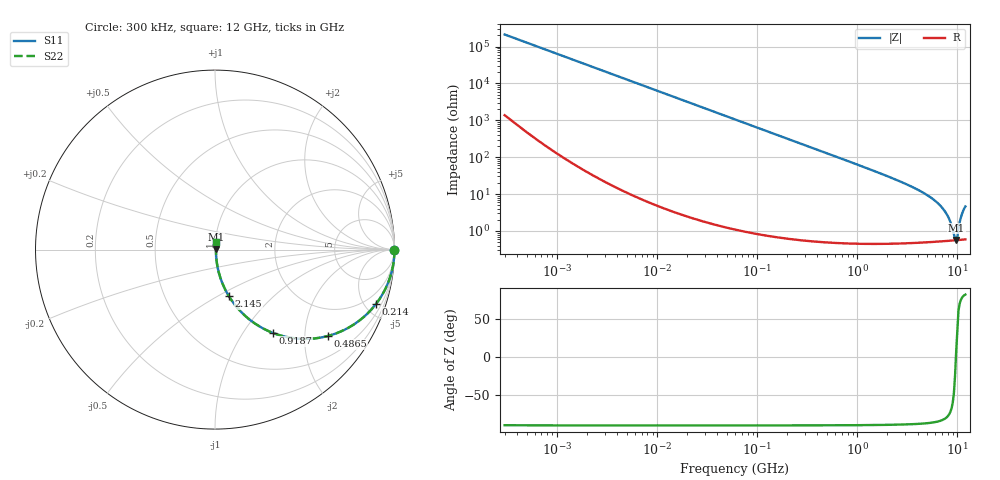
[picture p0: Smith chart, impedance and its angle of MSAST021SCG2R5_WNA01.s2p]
! MSAST021SCG2R5_WNA01  S-PARAMETER MODEL  ( General Type )
! Model Generated by TAIYO YUDEN Corporation (http://www.ty-top.com)
! Version 2.0
! TAIYO YUDEN Control No. 181101
! Copyright(c) 2015 TAIYO YUDEN CO.,LTD. All Rights Reserved.
! Product Description (link to TY-COMPAS)
! https://ds.yuden.co.jp/TYCOMPAS/or/detail?pn=MSAST021SCG2R5BWNA01&u=M
! Products Name : Multilayer Ceramic Capacitors
! Characteristics :
!  Capacitance : 2.5 pF , Rated Voltage : 25V , TCC : CG / C0G
!  Case Size : 0.25 x 0.125 / 0.0098 x 0.0049 [mm/inch] , Thickness : 0.125 / 0.0049 [mm/inch]
!  (Conditions: Temperature = 25 degC , DC Bias Current/Voltage = 0A / 0V)
! External Node Assignments :
!  1  o---| |---o  2
! GND o---------o GND
! Frequency Range : 0.3MHz  -  12000MHz  [ 401 STEP ]
# MHz S RI R 50
! Freq[MHz].  S11 Real  S11 Imag  S21 Real  S21 Imag  S12 Real  S12 Imag  S22 Real  S22 Imag
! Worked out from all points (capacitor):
!   401 points, 300 kHz to 12 GHz, reference 50 ohm
!   read as one part in series: C = 2.5 pF near 316.3 kHz
!   lowest |Z| = 566 mohm at 9.708 GHz (marker M1)
!   series resonance near 9.652 GHz, so ESL is about 110 pH
!   S11 on the Smith chart (normalised r, x): 300 kHz: open; 214 MHz: 1.01, -5.95; 486.5 MHz: 1.01, -2.61; 918.7 MHz: 1.01, -1.37; 2.145 GHz: 1.01, -0.56; 12 GHz: 1.01, +0.09
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0.3  1 -0.000471  3.28e-06 0.000471  3.28e-06 0.000471  1 -0.000471
1.769972  1 -0.00278  1.14e-05 0.00278  1.14e-05 0.00278  1 -0.00278
10.44266  0.9997 -0.0164  0.000281 0.0164  0.000281 0.0164  0.9997 -0.0164
60  0.9911 -0.0934  0.0089 0.0934  0.0089 0.0934  0.9911 -0.0934
213.9924  0.8979 -0.3018  0.1021 0.3018  0.1021 0.3018  0.8979 -0.3018
353.9943  0.7627 -0.424  0.2373 0.424  0.2373 0.424  0.7627 -0.424
486.4723  0.6297 -0.481  0.3703 0.481  0.3703 0.481  0.6297 -0.481
918.7169  0.3215 -0.4638  0.6785 0.4638  0.6785 0.4638  0.3215 -0.4638
1366.97  0.1748 -0.3749  0.8252 0.3749  0.8252 0.3749  0.1748 -0.3749
2088.533  0.0813 -0.2657  0.9187 0.2657  0.9187 0.2657  0.0813 -0.2657
2144.601  0.0773 -0.2592  0.9227 0.2592  0.9227 0.2592  0.0773 -0.2592
4050.141  0.021 -0.1261  0.979 0.1261  0.979 0.1261  0.021 -0.1261
6188.031  0.00868 -0.0597  0.9913 0.0597  0.9913 0.0597  0.00868 -0.0597
7064.448  0.00693 -0.0412  0.9931 0.0412  0.9931 0.0412  0.00693 -0.0412
7854.144  0.00606 -0.027  0.9939 0.027  0.9939 0.027  0.00606 -0.027
8503.825  0.00569 -0.0165  0.9943 0.0165  0.9943 0.0165  0.00569 -0.0165
9207.246  0.00555 -0.00603  0.9944 0.00603  0.9944 0.00603  0.00555 -0.00603
9454.42  0.00555 -0.00257  0.9944 0.00257  0.9944 0.00257  0.00555 -0.00257
9708.23  0.00558 0.000724  0.9944 -0.000724  0.9944 -0.000724  0.00558 0.000724
9968.853  0.00563 0.00385  0.9944 -0.00385  0.9944 -0.00385  0.00563 0.00385
11083.22  0.00653 0.0277  0.9935 -0.0277  0.9935 -0.0277  0.00653 0.0277
12000  0.00791 0.0451  0.9921 -0.0451  0.9921 -0.0451  0.00791 0.0451
